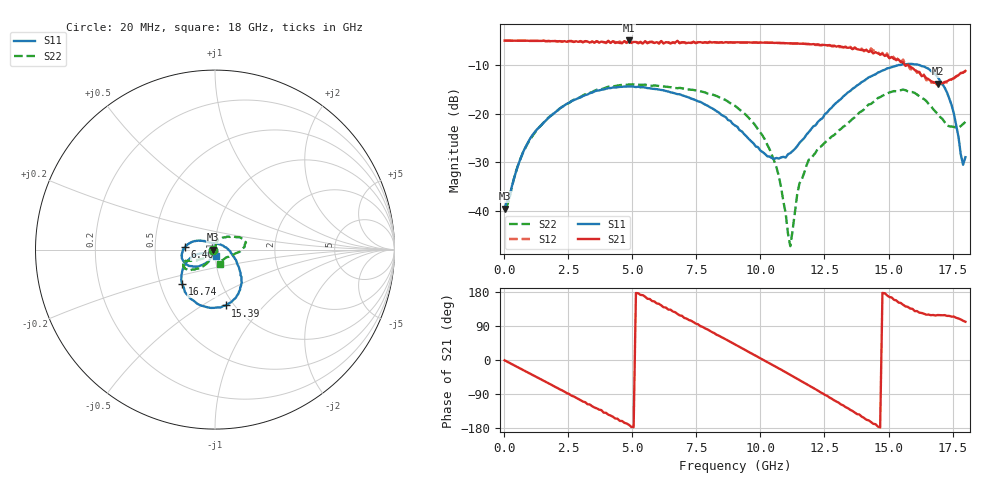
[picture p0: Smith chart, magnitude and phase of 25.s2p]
!Agilent Technologies,N5230A,US43500223,A.07.50.48
!Agilent N5230A: A.07.50.48
!Date: Sunday, January 10, 2016 17:39:42
!Correction: S11(Full 2 Port(1,2))
!S21(Full 2 Port(1,2))
!S12(Full 2 Port(1,2))
!S22(Full 2 Port(1,2))
!S2P File: Measurements: S11, S21, S12, S22:
# Hz S  dB  R 50
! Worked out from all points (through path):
!   201 points, 20 MHz to 18 GHz, reference 50 ohm
!   highest |S21| = -4.92 dB at 4.875 GHz (marker M1); lowest = -13.9 dB at 16.92 GHz (marker M2)
!   group delay of S21, straight-line fit = 100 ps
!   lowest |S11| = -39.6 dB at 20 MHz (marker M3), VSWR 1.02, Z = 49 - j0.0102 ohm
!   |S11| at or under -10 dB: start of sweep to 15.39 GHz; 16.21 GHz to end of sweep
!   |S22| runs from -47.3 to -14.0 dB; largest |S21 - S12| = 0.035
!   S11 on the Smith chart (normalised r, x): 20 MHz: 0.98, -0.00; 6.403 GHz: 0.71, +0.02; 15.39 GHz: 0.92, -0.63; 16.74 GHz: 0.65, -0.27; 18 GHz: 1.01, -0.07
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2e7  -39.58 -179.4  -4.95 -0.8  -4.94 -0.7  -39.28 -175.3
1.0988e9  -24.50 -116.6  -5.02 -39.1  -5.01 -39.1  -24.69 -114.7
2.1776e9  -18.92 -130.2  -5.07 -77.7  -5.06 -77.8  -18.95 -125.5
3.0766e9  -16.39 -141.3  -5.32 -109.6  -5.24 -109.5  -16.25 -135.0
4.8746e9  -14.40 -165.3  -4.92 -171.2  -5.09 -170.9  -14.00 -149.1
6.0433e9  -15.05 179.5  -5.44 148.1  -5.60 147.2  -14.32 -155.8
6.4029e9  -15.45 175.7  -5.35 133.2  -5.26 133.1  -14.51 -157.3
7.6615e9  -17.59 160.3  -5.27 89.2  -5.33 88.8  -15.41 -158.1
9.01e9  -22.45 140.3  -5.34 41.4  -5.33 41.1  -18.40 -151.0
1.04484e10  -29.16 93.4  -5.37 -12.2  -5.39 -12.6  -28.51 -133.4
1.0808e10  -29.04 70.8  -5.47 -25.3  -5.47 -25.7  -35.19 -132.2
1.11676e10  -28.13 48.9  -5.54 -39.2  -5.48 -40.0  -47.34 145.2
1.15272e10  -26.03 26.6  -5.60 -53.1  -5.58 -53.7  -34.38 83.9
1.20666e10  -22.64 1.6  -5.67 -74.2  -5.74 -74.5  -28.63 79.8
1.39545e10  -13.49 -45.9  -6.94 -149.5  -6.61 -150.3  -19.51 42.1
1.50333e10  -10.58 -68.7  -8.60 166.2  -8.49 165.6  -15.64 21.2
1.53929e10  -9.99 -79.1  -8.87 151.6  -8.42 148.8  -15.22 14.8
1.67414e10  -11.54 -133.7  -13.49 118.8  -13.66 119.2  -19.07 -12.7
1.69212e10  -12.49 -142.1  -13.86 118.6  -14.26 118.3  -20.07 -19.5
1.74606e10  -18.23 -164.1  -12.93 114.5  -12.94 114.1  -22.67 -47.2
1.79101e10  -30.56 -113.5  -11.58 103.6  -11.52 103.1  -22.16 -68.3
1.8e10  -28.99 -78.3  -11.19 101.0  -11.27 100.3  -21.72 -70.9
